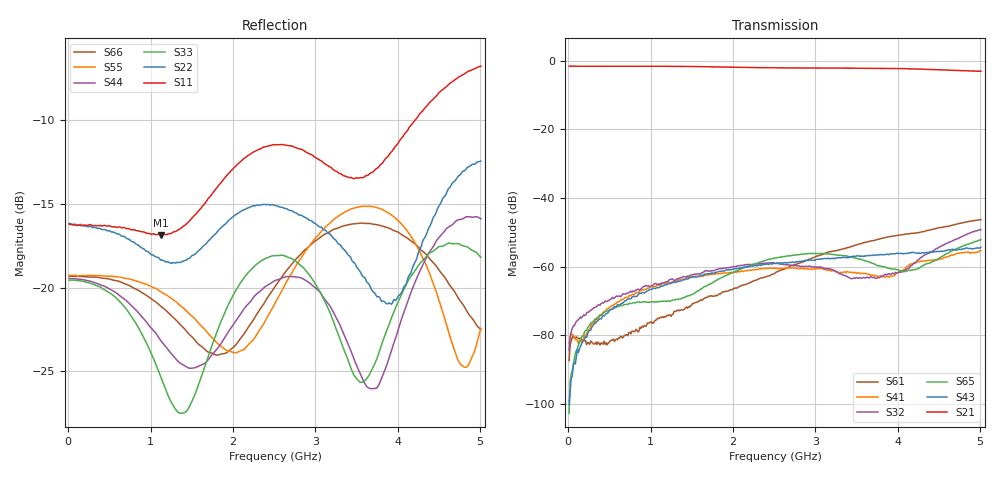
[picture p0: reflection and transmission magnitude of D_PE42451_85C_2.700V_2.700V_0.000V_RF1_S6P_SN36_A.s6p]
! Device ID: PE42451
! Serial: 36
! Insertion: A
! Temp: 85C
! VDD: 2.700
! Control_Hi: 100.000
! Control_Lo: 0.000
! Logic State: RF1
! Port 1: RFC
! Port 2: RF1
! Port 3: RF2
! Port 4: RF3
! Port 5: RF4
! Port 6: RF5
! V1 = 2.70
! V2 = 0.00
! V3 = 0.00
! V4 = 0.00
! IDD: 1.131390e-05
#  Hz  S  RI  R  50
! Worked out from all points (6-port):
!   401 points, 10 MHz to 5.01 GHz, reference 50 ohm
!   strongest paths, dB at 10 MHz, 1.26 GHz, 2.51 GHz, 3.76 GHz, 5.01 GHz:
!     S21: -1.6, -1.6, -2.1, -2.2, -3.1
!     S43: -100.4, -64.6, -59.1, -56.6, -54.4
!     S65: -102.8, -69.8, -57.5, -59.7, -52.2
!     S32: -84.4, -63.6, -59.1, -63.2, -49.2
!     S41: -82.4, -64.6, -60.5, -62.9, -55.3
!     S61: -87.4, -74.0, -62.0, -52.0, -46.3
!   lowest |S11| = -16.8 dB at 1.123 GHz (marker M1), VSWR 1.34, Z = 59 - j13 ohm
!   |S11| at or under -10 dB: start of sweep to 4.208 GHz
